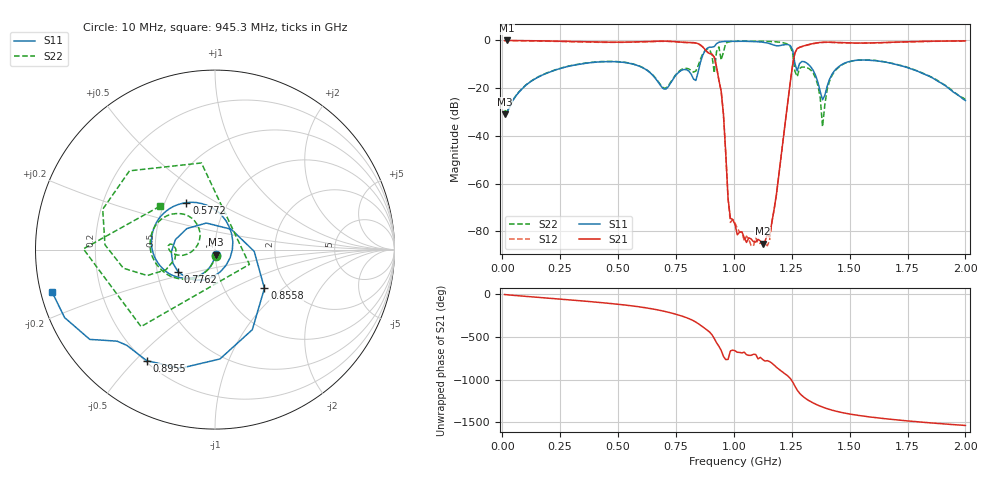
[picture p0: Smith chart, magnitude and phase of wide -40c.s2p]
!Agilent Technologies,E8363B,SG43030131,A.07.50.48
!Agilent E8363B: A.07.50.48
!Date: Monday, December 01, 2025 21:10:03
!Correction: S11(Full 2 Port(1,2))
!S21(Full 2 Port(1,2))
!S12(Full 2 Port(1,2))
!S22(Full 2 Port(1,2))
!S2P File: Measurements: S11, S21, S12, S22:
# Hz S  dB  R 50
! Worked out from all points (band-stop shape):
!   201 points, 10 MHz to 2 GHz, reference 50 ohm
!   highest |S21| = 0.01 dB at 19.95 MHz (marker M1); lowest = -85.2 dB at 1.124 GHz (marker M2)
!   |S21| within 3 dB of the highest: start of sweep to 868.4 MHz; 1.281 GHz to end of sweep
!   lowest |S11| = -30.9 dB at 10 MHz (marker M3), VSWR 1.06, Z = 50.2 - j2.84 ohm
!   |S11| at or under -10 dB: start of sweep to 330.8 MHz; 567.6 MHz to 853.6 MHz (286 MHz wide, 40.2 % of centre); 1.699 GHz to end of sweep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
!   |S22| runs from -36.2 to -0.3 dB; largest |S21 - S12| = 0.024
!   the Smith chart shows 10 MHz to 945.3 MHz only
!   S11 on the Smith chart (normalised r, x): 10 MHz: 1.00, -0.06; 577.1 MHz: 0.64, +0.37; 776.1 MHz: 0.64, -0.17; 855.8 MHz: 1.54, -0.76; 895.5 MHz: 0.21, -0.54; 945.3 MHz: 0.03, -0.13
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1e7  -30.92 -83.9  -0.02 -0.6  -0.07 -1.9  -29.29 -82.2
1.995e7  -30.15 -88.3  0.01 -3.4  -0.07 -4.4  -29.85 -91.0
3.483e8  -9.72 -166.9  -0.56 -76.2  -0.65 -76.3  -9.63 -163.5
5.7715e8  -10.27 121.3  -0.58 -139.6  -0.67 -139.7  -10.19 140.2
6.7665e8  -17.92 42.8  -0.29 175.9  -0.37 175.8  -17.67 130.4
7.7615e8  -12.39 -149.1  -0.71 106.1  -0.79 105.9  -12.04 -177.8
8.5575e8  -9.12 -38.1  -1.85 -0.4  -1.94 -0.5  -7.87 -159.1
8.9555e8  -2.78 -121.6  -5.52 -82.5  -5.59 -82.8  -3.77 137.4
9.254e8  -1.32 -144.4  -11.07 152.2  -11.16 152.0  -4.51 -133.9
9.453e8  -0.56 -165.3  -21.25 63.5  -21.32 63.2  -8.18 141.5
9.851e8  -0.35 165.6  -74.48 56.3  -76.27 49.0  -0.47 157.9
1.005e9  -0.35 153.4  -77.16 59.3  -76.55 58.2  -0.35 142.6
1.1244e9  -0.72 63.5  -85.20 -44.3  -84.48 -24.6  -0.34 78.4
1.1841e9  -2.22 -74.4  -64.29 -134.7  -64.65 -134.0  -0.57 36.5
1.2239e9  -1.68 169.3  -32.87 143.0  -32.98 142.8  -1.22 -12.2
1.2637e9  -9.69 77.1  -5.22 3.1  -5.32 3.1  -12.88 -122.3
1.29355e9  -8.81 111.2  -2.52 -106.6  -2.60 -106.7  -11.13 -143.5
1.3433e9  -12.64 73.3  -1.26 164.0  -1.34 163.8  -13.78 81.3
1.3831e9  -24.84 107.4  -0.75 116.7  -0.82 116.6  -36.18 -30.8
1.4428e9  -11.83 152.7  -0.83 67.1  -0.91 67.0  -12.11 153.4
1.67165e9  -9.37 77.4  -0.77 -25.1  -0.85 -25.4  -9.31 50.5
2e9  -25.13 69.0  -0.16 -99.3  -0.23 -99.4  -24.77 -86.7
